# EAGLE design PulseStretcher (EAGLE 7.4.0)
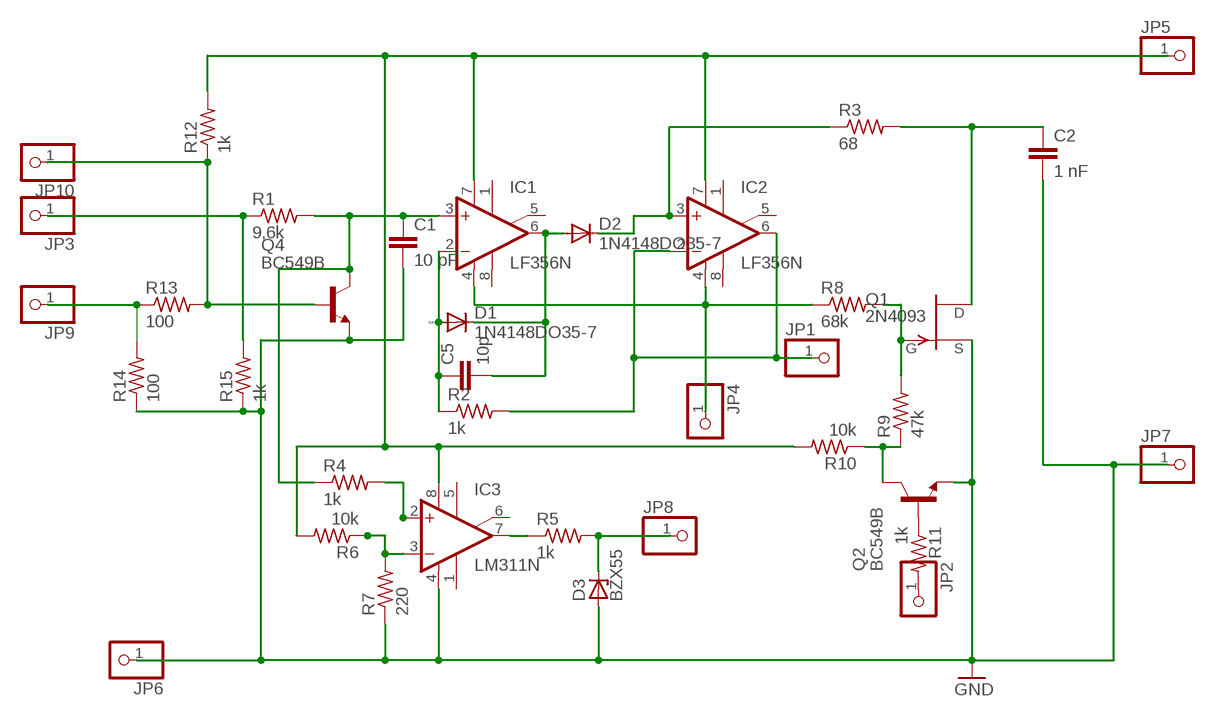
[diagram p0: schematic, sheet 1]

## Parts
C1  10 pF  C-EU050-024X044  [C050-024X044]
C2  1 nF  C-EU050-024X044  [C050-024X044]
C5  10p  C-EU050-024X044  [C050-024X044]
D1  1N4148DO35-7  [DO35-7]
D2  1N4148DO35-7  [DO35-7]
D3  BZX55  [DO35Z10]
IC1  LF356N  [DIL08]
IC2  LF356N  [DIL08]
IC3  LM311N  [DIL08]
JP1  PINHD-1X1  [1X01]
JP2  PINHD-1X1  [1X01]
JP3  PINHD-1X1  [1X01]
JP4  PINHD-1X1  [1X01]
JP5  PINHD-1X1  [1X01]
JP6  PINHD-1X1  [1X01]
JP7  PINHD-1X1  [1X01]
JP8  PINHD-1X1  [1X01]
JP9  PINHD-1X1  [1X01]
JP10  PINHD-1X1  [1X01]
Q1  2N4093  [TO18]
Q2  BC549B  [TO92-EBC]
Q4  BC549B  [TO92-EBC]
R1  9,6k  R-US_0204/5  [0204/5]
R2  1k  R-US_0204/5  [0204/5]
R3  68  R-US_0204/5  [0204/5]
R4  1k  R-US_0204/5  [0204/5]
R5  1k  R-US_0204/5  [0204/5]
R6  10k  R-US_0204/5  [0204/5]
R7  220  R-US_0204/5  [0204/5]
R8  68k  R-US_0204/5  [0204/5]
R9  47k  R-US_0204/5  [0204/5]
R10  10k  R-US_0204/5  [0204/5]
R11  1k  R-US_0204/5  [0204/5]
R12  1k  R-US_0204/5  [0204/5]
R13  100  R-US_0204/5  [0204/5]
R14  100  R-US_0204/5  [0204/5]
R15  1k  R-US_0204/5  [0204/5]

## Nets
GND: C1.2 C2.2 D3.A IC3.4(V-) JP6.1 JP7.1 Q1.1(S) Q2.E Q4.E R7.1 R14.1 R15.1
N$1: C1.1 IC1.3(+IN) Q4.C R1.2 R4.1
N$2: C5.1 D1.A IC1.2(-IN) R2.1
N$3: C2.1 Q1.2(D) R3.2
N$4: D2.C IC2.3(+IN) R3.1
N$5: IC2.2(-IN) IC2.6(OUT) JP1.1 R2.2
N$6: IC3.2(+IN) R4.2
N$7: C5.2 D1.C D2.A IC1.6(OUT)
N$8: Q1.3(G) R8.2 R9.2
N$9: JP3.1 R1.1 R15.2
N$10: Q2.B R11.1
N$12: IC3.7(OUT) R5.1
N$13: IC1.4(V-) IC2.4(V-) JP4.1 R8.1
N$14: Q2.C R9.1 R10.1
N$15: IC3.3(-IN) R6.1 R7.2
N$16: JP2.1 R11.2
N$17: D3.C JP8.1 R5.2
N$18: JP10.1 Q4.B R12.1 R13.2
N$19: JP9.1 R13.1 R14.2
N$20: IC1.7(V+) IC2.7(V+) IC3.8(V+) JP5.1 R6.2 R10.2 R12.2
Unconnected: IC1.1(ON1) IC1.5(ON2) IC1.8(OPT) IC2.1(ON1) IC2.5(ON2) IC2.8(OPT) IC3.1(GND) IC3.5(ON) IC3.6(ON/STR)

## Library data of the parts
C1 C2 C5 = rcl:C-EU: CAPACITOR, European symbol
D1 D2 = diode:1N4148: DIODE
D3 = diode:BZX55: Z DIODE
IC1 IC2 = linear:LF356: OP AMP
IC3 = linear:LM311: COMPARATOR
JP1-JP10 = pinhead:PINHD-1X1: PIN HEADER
Q1 = transistor-fet:2N4093: N-Channel Junction FET
Q2 Q4 = transistor-npn:BC549*: NPN Transistor
R1-R15 = rcl:R-US_: RESISTOR, American symbol

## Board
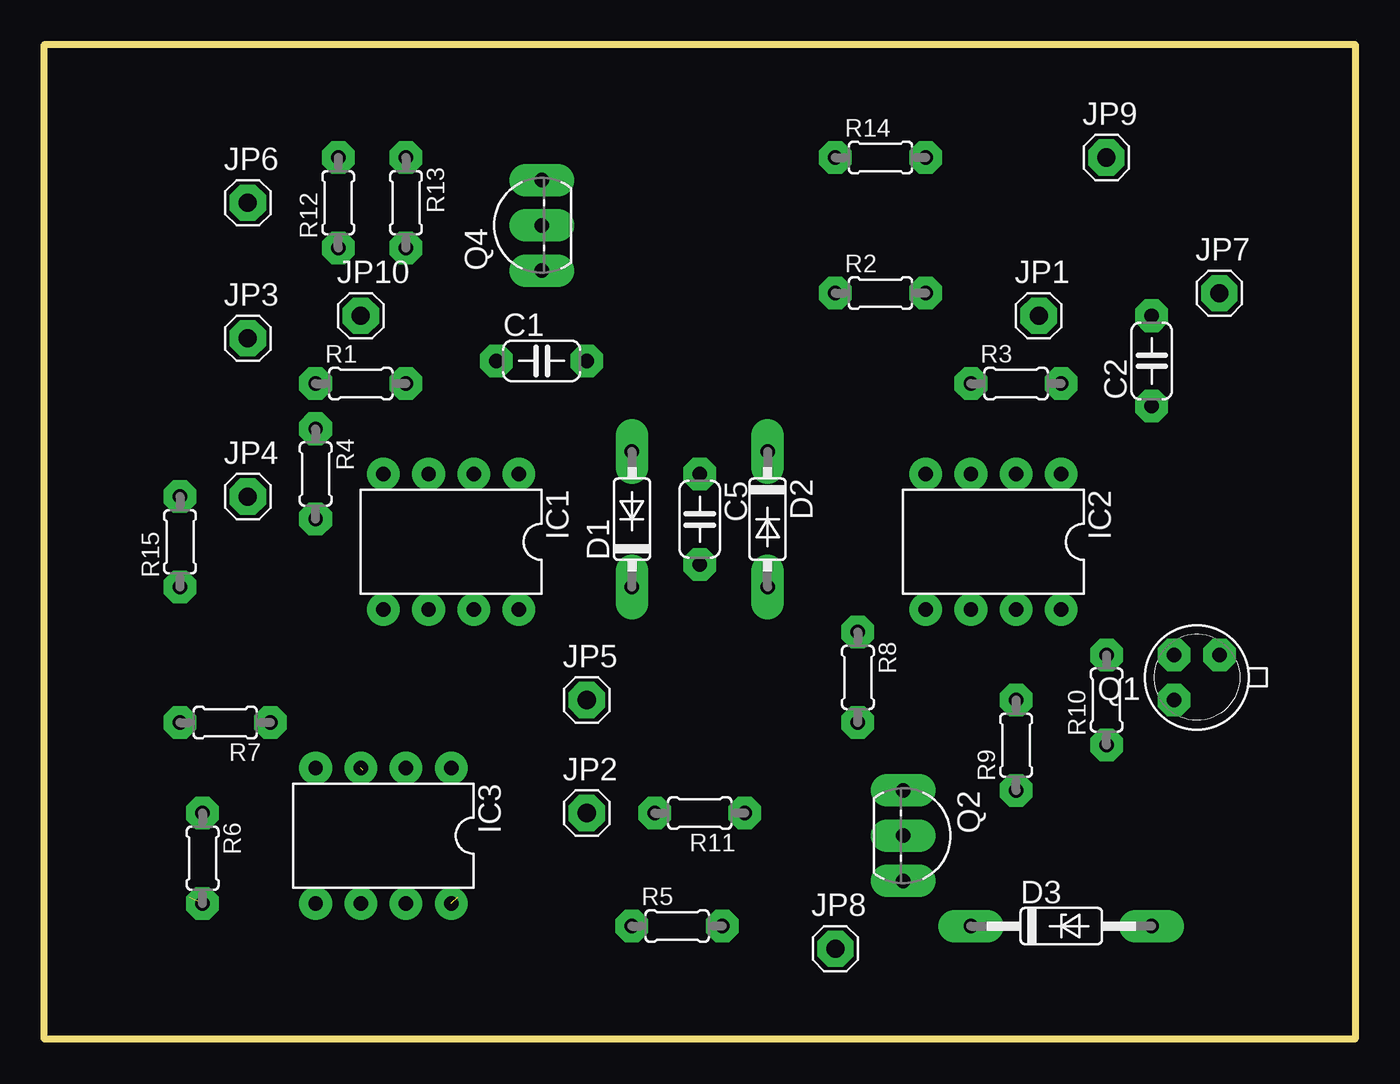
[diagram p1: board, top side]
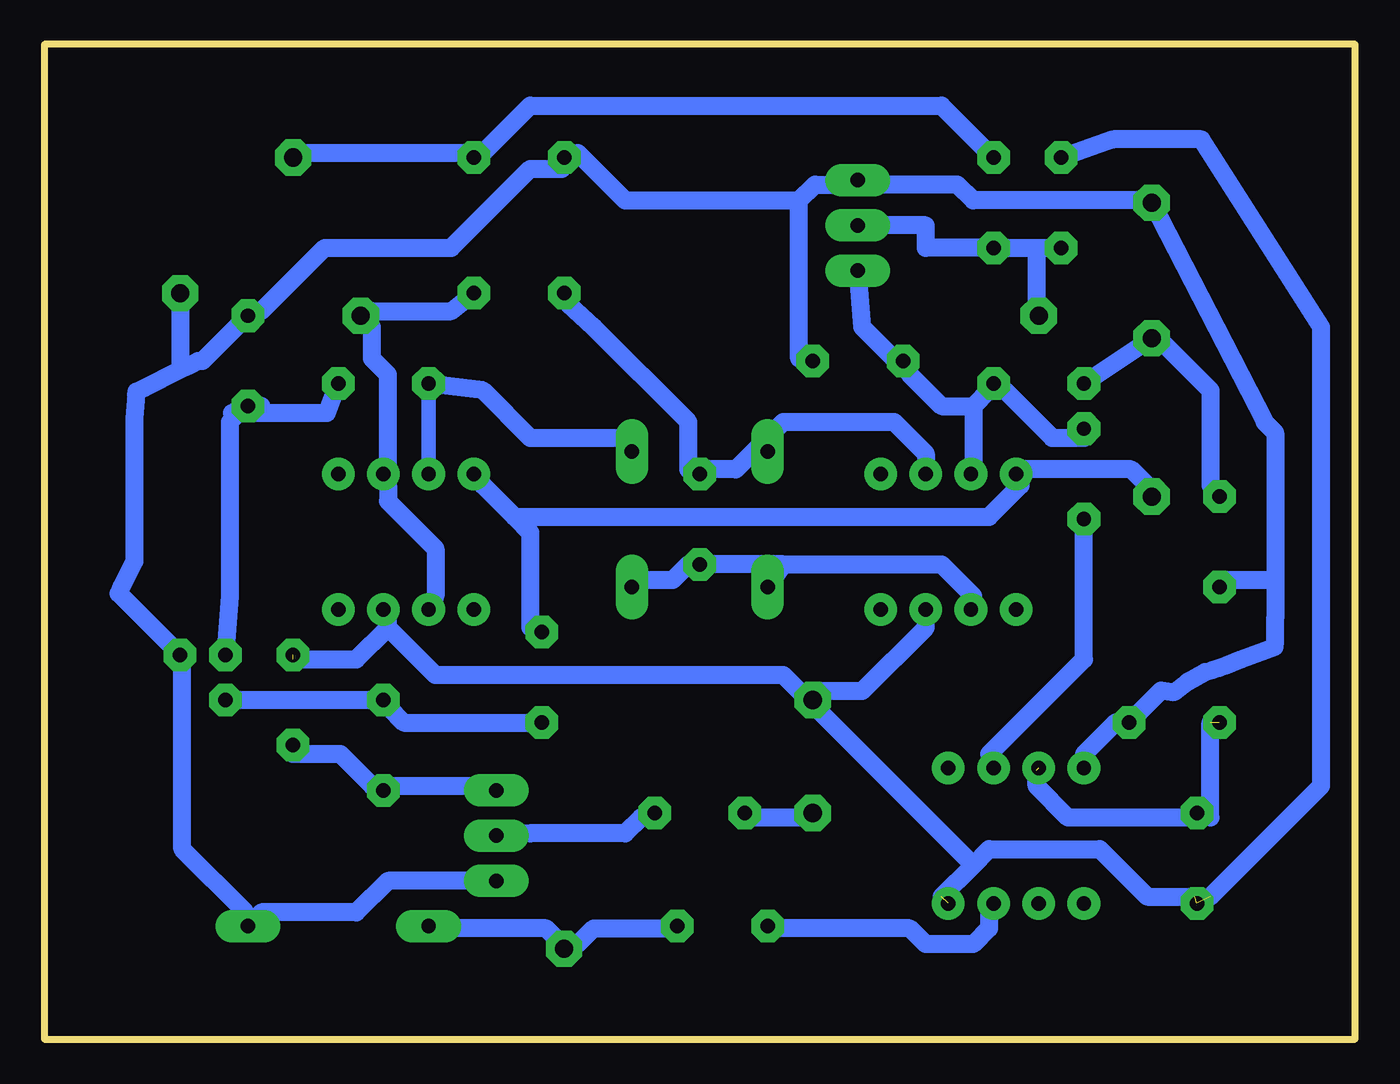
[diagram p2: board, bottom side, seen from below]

Size 73.66 x 55.88 mm. Coordinates in mm from the lower left corner, seen from the top.
Outline: 0,55.88 73.66,55.88 73.66,0 0,0 0,55.88
Copper layers (1*16): Top 0.035mm / dielectric 1.5mm / Bottom 0.035mm
Design rules "default *": minimum track width 40mil, minimum drill 24mil, track to track 30mil, track to pad 30mil, pad to pad 8mil, via to via 8mil, smd to smd 8mil, copper to edge 40mil, drill to drill 8mil, minimum pad ring 20mil, minimum via ring 8mil, stop-mask expansion 4mil, vias tented up to drill 0mil, thermal gap 10mil

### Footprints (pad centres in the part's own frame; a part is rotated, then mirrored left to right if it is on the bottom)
C050-024X044 = drill 0.813 octagon: 1 -2.54,0; 2 2.54,0
DO35-7 = drill 0.813 long: A 3.81,0; C -3.81,0
DO35Z10 = drill 0.813 long: A 5.08,0; C -5.08,0
DIL08 = drill 0.813 pad 1.27: 1 -3.81,-3.81; 2 -1.27,-3.81; 3 1.27,-3.81; 4 3.81,-3.81; 5 3.81,3.81; 6 1.27,3.81; 7 -1.27,3.81; 8 -3.81,3.81
1X01 = drill 1.016 octagon: 1 0,0
TO18 = drill 0.813 octagon: 1 -1.27,-1.27; 2 1.27,-1.27; 3 1.27,1.27
TO92-EBC = drill 0.813 long: B 0,-1.27; C -2.54,-1.27; E 2.54,-1.27
0204/5 = drill 0.813 octagon: 1 -2.54,0; 2 2.54,0

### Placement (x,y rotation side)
C1  27.94,38.1 0 top
C2  62.23,38.1 90 top
C5  36.83,29.21 270 top
D1  33.02,29.21 90 top
D2  40.64,29.21 270 top
D3  57.15,6.35 0 top
IC1  22.86,27.94 180 top
IC2  53.34,27.94 180 top
IC3  19.05,11.43 180 top
JP1  55.88,40.64 0 top
JP2  30.48,12.7 0 top
JP3  11.43,39.37 0 top
JP4  11.43,30.48 0 top
JP5  30.48,19.05 0 top
JP6  11.43,46.99 0 top
JP7  66.04,41.91 0 top
JP8  44.45,5.08 0 top
JP9  59.69,49.53 0 top
JP10  17.78,40.64 0 top
Q1  64.77,20.32 180 top
Q2  49.53,11.43 270 top
Q4  26.67,45.72 90 top
R1  17.78,36.83 0 top
R2  46.99,41.91 0 top
R3  54.61,36.83 0 top
R4  15.24,31.75 270 top
R5  35.56,6.35 0 top
R6  8.89,10.16 270 top
R7  10.16,17.78 180 top
R8  45.72,20.32 270 top
R9  54.61,16.51 90 top
R10  59.69,19.05 90 top
R11  36.83,12.7 180 top
R12  16.51,46.99 90 top
R13  20.32,46.99 270 top
R14  46.99,49.53 0 top
R15  7.62,27.94 90 top

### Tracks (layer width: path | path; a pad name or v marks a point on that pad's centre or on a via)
GND
  Bottom 1.016: IC3.4 15.24,16 13.46,17.78 R7.1 10.89,19.59 10.16,19.49 9.39,20.08 8.44,20.61 8,20.74 7.65,20.85 7.24,20.99 6.42,21.33 4.51,22.03 4.49,22.34 4.48,23.62 4.48,25.78 | Q2.E 54.36,8.89 56.13,7.11 61.47,7.11 D3.A 62.36,7.11 65.91,10.67 65.91,21.34 Q1.1 69.49,25.04 69.33,25.42 68.6,26.84 68.6,34.88 68.51,36.22 68.5,36.37 68.05,36.59 66.13,37.57 66.04,37.61 | JP7.1 66.04,37.61 | 66.04,37.61 65.62,37.81 65.5,37.86 65.02,38.1 64.77,38.1 C2.2 61.47,40.89 57.91,44.45 50.8,44.45 46.36,48.89 44.58,48.89 R14.1 43.69,49.78 41.02,47.12 31.24,47.12 | 4.48,25.78 4.48,34.08 5.06,34.65 5.08,34.67 JP6.1 11.68,47.12 21.46,47.12 22.35,48.01 27.69,48.01 Q4.E 28.57,48.01 30.35,48.01 31.24,47.12 | 4.48,25.78 7.24,25.78 R15.1 | 31.24,47.12 31.24,38.23 C1.2
N$1
  Bottom 1.016: Q4.C 27.69,40 25.91,38.23 C1.1 25.02,37.34 23.24,35.56 21.46,35.56 | 21.46,35.56 21.46,32 IC1.3 | 21.46,35.56 20.57,36.45 R1.2 19.69,36.45 17.02,33.78 15.24,33.78 R4.1
N$2
  Bottom 1.016: 33.02,33.78 34.8,32 36.58,32 C5.1 37.47,32 37.47,34.67 42.8,40 44.2,41.27 R2.1 | IC1.2 24.13,32.89 25.91,34.67 32.13,34.67 33.02,33.78 | 33.02,33.78 D1.A
N$3
  Bottom 1.016: R3.2 57.79,35.18 63.12,35.18 61.47,35.56 C2.1 62.36,35.56 63.25,34.67 63.25,24.89 Q1.2
N$4
  Bottom 0.813: R3.1 IC2.3
  Bottom 1.016: D2.C 41.02,33.78 46.36,33.78 49.02,36.45 R3.1
N$5
  Bottom 1.016: IC2.6 51.69,24.89 51.69,27.56 54.36,30.23 54.36,31.12 IC2.2 54.36,32 54.36,37.34 55.24,38.23 55.24,40 JP1.1 55.24,40.89 50.8,40.89 R2.2
N$6
  Bottom 1.016: R4.2 15.24,21.34 20.57,16 IC3.2
N$7
  Bottom 1.016: D2.A 40.13,25.78 38.35,25.78 37.47,26.67 C5.2 32.13,26.67 | 32.13,26.67 23.24,26.67 21.46,24.89 IC1.6 | 32.13,26.67 33.02,25.78 D1.C 32.13,26.67
N$8
  Bottom 1.016: R8.2 53.47,17.78 54.36,18.67 R9.2 Q1.3
N$9
  Bottom 1.016: R15.2 8.13,31.12 8.13,36.45 10.8,39.12 JP3.1 R1.1
N$10
  Bottom 1.016: Q2.B 46.36,11.56 41.02,11.56 40.13,12.45 R11.1
N$12
  Bottom 1.016: R5.1 33.02,6.22 25.02,6.22 24.13,5.33 21.46,5.33 20.57,6.22 20.57,7.11 IC3.7
N$13
  Bottom 1.016: JP4.1 11.68,31.12 12.57,32 18.8,32 IC1.4 18.8,31.12 20.57,29.34 47.24,29.34 | 47.24,29.34 49.02,31.12 IC2.4 | 47.24,29.34 46.36,28.45 46.36,23.11 R8.1
N$14
  Bottom 1.016: R10.1 59.69,16 57.02,16 55.24,14.22 R9.1 54.36,14.22 47.24,14.22 Q2.C
N$15  (2 unrouted)
  Bottom 1.016: 8.13,17.78 8.13,12.45 R6.1 9.02,12.45 16.13,12.45 17.91,14.22 17.91,15.11
N$16
  Bottom 1.016: R11.2 33.91,12.45 31.24,12.45 JP2.1
N$17
  Bottom 1.016: R5.2 38.35,6.22 42.8,6.22 43.69,5.33 JP8.1 44.58,5.33 45.47,6.22 51.69,6.22 D3.C
N$18
  Bottom 1.016: 17.91,44.45 R13.2 24.13,44.45 24.13,45.72 Q4.B | 17.91,44.45 R12.1 | 17.91,44.45 17.91,40.89 JP10.1
N$19
  Bottom 1.016: JP9.1 59.69,49.78 49.91,49.78 R14.2 49.02,49.78 46.36,52.45 23.24,52.45 R13.1
N$20  (4 unrouted)
  Bottom 1.016: 9.02,8 11.68,8 14.35,10.67 20.57,10.67 21.46,9.78 | 23.24,8 21.46,9.78 | IC1.7 24.13,23.11 27.69,19.56 30.35,19.56 JP5.1 | 21.46,9.78 30.35,18.67 JP5.1 | 54.36,23.11 54.36,24 IC2.7 | 54.36,23.11 56.13,21.34 59.69,21.34 | 54.36,23.11 51.69,20.45 32.13,20.45 31.24,19.56 JP5.1 | 8.13,8 1.91,14.22 1.91,40 8.64,50.55 13.59,50.55 R12.2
